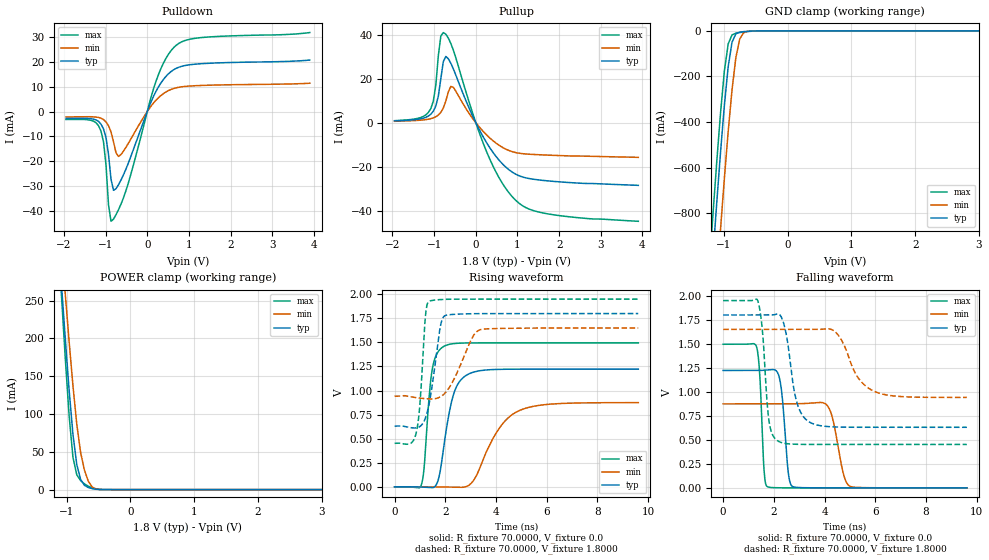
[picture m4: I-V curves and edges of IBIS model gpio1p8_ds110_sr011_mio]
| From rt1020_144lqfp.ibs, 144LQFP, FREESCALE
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[Model] gpio1p8_ds110_sr011_mio
|   Model gpio1p8_ds110_sr011_mio
| This model was characterised for following simulation conditions:
| External (pad) voltage:
|   - Typ: 1.8V,   - Min: 1.65V,   - Max: 1.95V
| Library cells for typ/min/max conditions are connected as defined below:
|  pad - External Pad
|  ipp_do - Core Input
|  ipp_obe - Output Buffer Enable
|  esd_boost - ovdd
|  ipp_dse0 - vssi
|  ipp_dse1 - vddi
|  ipp_dse2 - vddi
|  ipp_fsel0 - vddi
|  ipp_fsel1 - vddi
|  ipp_ina - ipp_ina
|  ipp_ind - ipp_ind
|  ipp_pwr_stable - vddi
|  ipp_sre - vssi
|  ovdd - ovdd
|  ovss - ovss
|  vddi - vddi
|  vssi - vssi
| All other pins connected to ground
Model_type I/O
Polarity   Non-Inverting
Enable   Active-High
Vinl =   0.5400V
Vinh =   1.2600V
Vmeas =  0.9000V
Cref =   0.0F
Rref =   70.0000
Vref =   0.9000V
C_comp   1.2573pF   1.2208pF   1.3056pF
|C_comp_pullup   0.6440pF   0.6611pF   0.6285pF
|C_comp_pulldown   0.5474pF   0.5788pF   0.5258pF
[Model Spec]
| variable   typ   min   max
Vinh   1.2600V   1.1550V   1.3650V
Vinl   0.5400V   0.4950V   0.5850V
S_overshoot_high   1.8000V   1.6500V   1.9500V
S_overshoot_low   0.0V   0.0V   0.0V
Vmeas   0.9000V   0.8250V   0.9750V
Vref   0.9000V   0.8250V   0.9750V
Cref   0.0F   0.0F   0.0F
Rref   70.0000   70.0000   70.0000
[Temperature Range]   25.0000   0.1050k   -20.0000
[Voltage Range]   1.8000V   1.6500V   1.9500V
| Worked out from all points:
|   slope of the pulldown table from 0 to 0.27 V, typ, clamps not added: 27.2 ohm
|   slope of the pullup table from 0 to 0.27 V, typ, clamps not added: 28.7 ohm
|   GND clamp passes 1 mA (typ) near -0.55 V on its own axis
|   POWER clamp passes 1 mA (typ) near -0.58 V on its own axis
|   rising waveform, R_fixture 70.0000, V_fixture 0.0: 20-80 % time 499ps typ, 1.09ns min, 276ps max; typ from 0 V to 1.22 V
|   rising waveform, R_fixture 70.0000, V_fixture 1.8000: 20-80 % time 381ps typ, 712ps min, 219ps max; typ from 0.631 V to 1.8 V
|   falling waveform, R_fixture 70.0000, V_fixture 0.0: 20-80 % time 217ps typ, 377ps min, 149ps max; typ from 1.22 V to 0 V
|   falling waveform, R_fixture 70.0000, V_fixture 1.8000: 20-80 % time 425ps typ, 800ps min, 238ps max; typ from 1.8 V to 0.631 V
[Pulldown]
|Voltage   I(typ)   I(min)   I(max)
-1.95V    -2.794mA   -2.176mA   -3.212mA
-1.29V    -3.073mA   -2.149mA   -3.876mA
-1.11V    -5.06mA    -2.697mA   -7.882mA
-990mV    -10.46mA   -4.192mA   -21.47mA
-930mV    -17.18mA   -5.69mA    -37.39mA
-870mV    -27.13mA   -8.178mA   -44mA
-810mV    -31.59mA   -12.14mA   -43.11mA
-690mV    -29.33mA   -18mA      -39.34mA
210mV     8.092mA    4.542mA    12.13mA
630mV     16.7mA     9.196mA    25.53mA
1.23V     19.07mA    10.39mA    29.5mA
3.9V      20.61mA    11.33mA    31.63mA
[Pullup]
|Voltage   I(typ)   I(min)   I(max)
-1.95V    820uA      630uA      920uA
-1.08V    3.846mA    1.832mA    6.417mA
-960mV    7.572mA    2.692mA    17.07mA
-900mV    12.06mA    3.465mA    30.37mA
-840mV    19.96mA    4.676mA    39.39mA
-780mV    27.77mA    6.655mA    40.96mA
-720mV    30.1mA     9.856mA    40.22mA
-540mV    24.49mA    16.07mA    33.02mA
240mV     -8.497mA   -5.208mA   -12.33mA
960mV     -23.42mA   -13.6mA    -35.32mA
1.74V     -26.47mA   -14.75mA   -41.48mA
3.9V      -28.48mA   -15.75mA   -44.82mA
[GND_clamp]
|Voltage   I(typ)   I(min)   I(max)
-1.95V    -4.191A    -4.477A    -4.042A
-1.23V    -1.234A    -1.577A    -1.052A
-1.17V    -993.2mA   -1.338A    -811.1mA
-1.11V    -758.1mA   -1.102A    -578.5mA
-1.05V    -533.7mA   -870.8mA   -361.6mA
-990mV    -328mA     -648.8mA   -176.9mA
-930mV    -157.5mA   -441.8mA   -57.56mA
-870mV    -50.13mA   -259.5mA   -18.17mA
-810mV    -13.28mA   -118mA     -10.41mA
-750mV    -5.921mA   -36.52mA   -7.502mA
-630mV    -2.275mA   -2.653mA   -3.283mA
3.9V      0A         0A         0A
[POWER_clamp]
|Voltage   I(typ)   I(min)   I(max)
-1.95V    1.356A     1.328A     1.514A
-1.08V    270.6mA    322.7mA    256.8mA
-1.02V    199mA      258.1mA    173mA
-960mV    131.2mA    195.7mA    97.36mA
-900mV    72.67mA    137.2mA    42.48mA
-840mV    32.99mA    86.34mA    19.5mA
-780mV    13.32mA    48.87mA    11.87mA
-720mV    5.671mA    25.66mA    7.515mA
-660mV    2.793mA    11.19mA    4.477mA
-600mV    1.289mA    3.449mA    2.334mA
-480mV    122.1uA    182.3uA    260.9uA
3.9V      0A         0A         0A
[Ramp]
| variable   typ   min   max
dV/dt_r  0.7336/0.4990n   0.5247/1.0853n   0.8973/0.2756n
dV/dt_f  0.7016/0.4254n   0.4252/0.7998n   0.8988/0.2377n
R_load = 70.0000
[Rising Waveform]
R_fixture= 70.0000
V_fixture= 0.0
V_fixture_min= 0.0
V_fixture_max= 0.0
|time   V(typ)   V(min)   V(max)
0s        378.5pV    3.584nV    765.1pV
1.061ns   -2.328mV   172.5uV    24.49mV
1.161ns   -3.739mV   155.2uV    188mV
1.477ns   -8.889mV   -166.4uV   1.207V
1.722ns   72.84mV    -923.1uV   1.405V
1.926ns   391.8mV    -1.929mV   1.457V
2.367ns   993.7mV    -4.577mV   1.489V
2.992ns   1.181V     29.38mV    1.495V
4.875ns   1.222V     786.8mV    1.496V
9.61ns    1.223V     874.5mV    1.496V
[Rising Waveform]
R_fixture= 70.0000
V_fixture= 1.8000
V_fixture_min= 1.6500
V_fixture_max= 1.9500
|time   V(typ)   V(min)   V(max)
0s        630.7mV    941.3mV    451.9mV
611.3ps   615.5mV    936.7mV    447.7mV
848.2ps   611.8mV    926.4mV    554.7mV
997.4ps   626.2mV    921.4mV    851.9mV
1.226ns   720.6mV    915.2mV    1.799V
1.371ns   875.1mV    912.7mV    1.929V
1.802ns   1.662V     934.4mV    1.945V
2.008ns   1.781V     978.9mV    1.948V
3.346ns   1.799V     1.63V      1.95V
9.61ns    1.8V       1.65V      1.95V
[Falling Waveform]
R_fixture= 70.0000
V_fixture= 0.0
V_fixture_min= 0.0
V_fixture_max= 0.0
|time   V(typ)   V(min)   V(max)
0s        1.223V     874.6mV    1.496V
1.326ns   1.223V     874.4mV    1.462V
1.445ns   1.223V     874.4mV    1.171V
1.612ns   1.224V     874.4mV    187.8mV
1.739ns   1.226V     874.4mV    13.19mV
2.229ns   1.133V     874.5mV    747.8uV
2.741ns   13.3mV     875.1mV    130.3uV
4.122ns   119.5uV    851.7mV    11.97uV
5.019ns   22.59uV    14.45mV    2.939uV
9.61ns    -529.9nV   477.5nV    -227nV
[Falling Waveform]
R_fixture= 70.0000
V_fixture= 1.8000
V_fixture_min= 1.6500
V_fixture_max= 1.9500
|time   V(typ)   V(min)   V(max)
0s        1.8V       1.65V      1.95V
1.363ns   1.8V       1.65V      1.95V
1.549ns   1.8V       1.65V      1.638V
1.806ns   1.8V       1.65V      701.2mV
2.182ns   1.81V      1.65V      484.7mV
2.903ns   894.2mV    1.65V      453.6mV
3.427ns   681.4mV    1.65V      452.1mV
4.468ns   633.8mV    1.612V     451.9mV
5.951ns   630.7mV    1.006V     451.9mV
9.61ns    630.7mV    941.4mV    451.9mV
